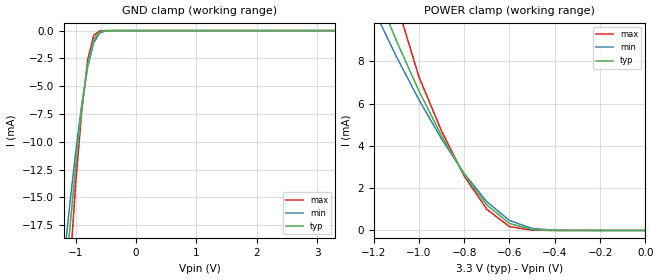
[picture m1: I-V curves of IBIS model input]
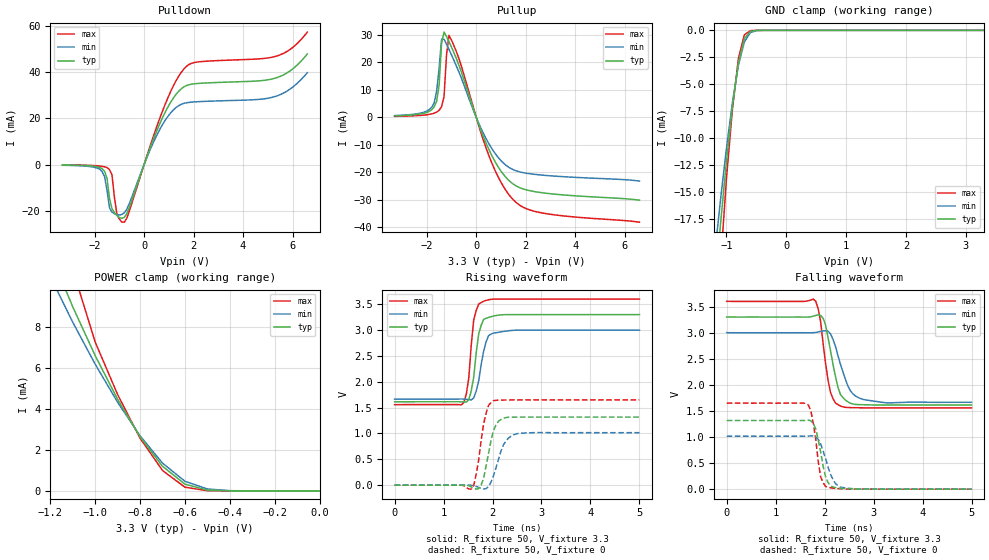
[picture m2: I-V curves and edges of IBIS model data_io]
| SOJ  Package & Industrial  operation.
[IBIS Ver]   3.2
[Comment Char]   |_char
[File name]   as7c3256a_soji.ibs
[File Rev]   1.0
[Date]   May 19, 2004 2:59:33 PM
[Source]
Alliance Semiconductor Corporation
[Notes]
This model  is for SOJ package & Industrial operation.
[Disclaimer]
Data is for modeling purpose only and is not guaranted.
This IBIS model is provided on an "AS IS" basis and Alliance Semiconductor makes
absolutely no warranty with respect to the information contained
herein.The entire risk as to quality and performance
is with the Customer. ACCORDINGLY, IN NO EVENT SHALL THE COMPANY BE
LIABLE FOR ANY DAMAGES, WHETHER IN CONTRACT OR TORT,INCLUDING ANY
LOST PROFITS OR OTHER INCIDENTAL, CONSEQUENTIAL, EXEMPLARY, OR
PUNITIVE DAMAGES ARISING OUT OF THE USE OR APPLICATION OF THE IBIS
model provided in this package.
[Copyright]
Alliance Semiconductor Corporation
| SOJ Package & Industrial  operation.
[Component]   AS7C3256A_SOJI
Si_location Pin
Timing_location Pin
[Manufacturer]   Alliance Semiconductor Corporation
[Package]
R_pkg   158.885m   88.47m   229.3m
L_pkg   7.1455nH   4.457nH   9.834nH
C_pkg   1.118pF   0.777pF   1.459pF
[Pin] signal_name   model_name
1   A14   input
2   A12   input
3   A7   input
4   A6   input
5   A5   input
6   A4   input
7   A3   input
8   A2   input
9   A1   input
10   A0   input
11   IO0   data_io
12   IO1   data_io
13   IO2   data_io
14   GND   GND
15   IO3   data_io
16   IO4   data_io
17   IO5   data_io
18   IO6   data_io
19   IO7   data_io
20   NCE   input
21   A10   input
22   NOE   input
23   A11   input
24   A9   input
25   A8   input
26   A13   input
27   NWE   input
28   VCC   POWER
| Models and submodels in the file (2): input (Input), data_io (I/O)
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[Model]   input
Model_type Input
Vinh=2V
Vinl=0.8V
C_comp   4pF   4pF   4pF
[Model Spec]
[Temperature Range] 25   85   -40
[Voltage Range]   3.3   3.0   3.6
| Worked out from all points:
|   GND clamp passes 1 mA (typ) near -0.71 V on its own axis
|   POWER clamp passes 1 mA (typ) near -0.68 V on its own axis
[GND Clamp]
-3.3V     -7.098A    -6.841A    -8.051A
-1.2V     -24.5mA    -21.03mA   -71.59mA
-1.1V     -18.08mA   -15.8mA    -21.91mA
-1V       -12.19mA   -10.98mA   -13.83mA
-900mV    -7.049mA   -6.709mA   -7.353mA
-800mV    -3.052mA   -3.264mA   -2.619mA
-700mV    -776.2uA   -1.076mA   -424.2uA
-600mV    -102uA     -214uA     -28.92uA
-500mV    -8.916uA   -29.72uA   -1.118uA
-400mV    -568.8nA   -3.277uA   -28.76nA
3.3V      81.27pA    1.281uA    71.95pA
[POWER Clamp]
-3.3V     7.097A     6.84A      8.051A
-1.2V     11.62mA    10.47mA    61.3mA
-1.1V     8.99mA     8.237mA    10.82mA
-1V       6.605mA    6.189mA    7.271mA
-900mV    4.474mA    4.328mA    4.704mA
-800mV    2.643mA    2.691mA    2.576mA
-700mV    1.205mA    1.359mA    1.001mA
-600mV    329.9uA    471.6uA    181.9uA
-500mV    42.94uA    94.79uA    11.57uA
-400mV    3.493uA    12.38uA    421.4nA
0V        81.27pA    182.3pA    86.4pA
[Model]   data_io
Model_type I/O
Enable Active-High
Polarity Non-Inverting
Vinh=2V
Vinl=0.8V
Vref=1.72V
Vmeas=1.5V
Rref=168
Cref=30pF
C_comp   4pF   4pF   4pF
[Temperature Range] 25   85   -40
[Voltage Range]   3.3   3.0   3.6
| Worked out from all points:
|   slope of the pulldown table from 0 to 0.495 V, typ, clamps not added: 34.8 ohm
|   slope of the pullup table from 0 to 0.495 V, typ, clamps not added: 43.5 ohm
|   GND clamp passes 1 mA (typ) near -0.71 V on its own axis
|   POWER clamp passes 1 mA (typ) near -0.68 V on its own axis
|   falling waveform, R_fixture 50, V_fixture 3.3: 20-80 % time 216ps typ, 278ps min, 176ps max; typ from 3.3 V to 1.61 V
|   falling waveform, R_fixture 50, V_fixture 0: 20-80 % time 170ps typ, 221ps min, 146ps max; typ from 1.32 V to 0.002 V
|   rising waveform, R_fixture 50, V_fixture 3.3: 20-80 % time 139ps typ, 163ps min, 117ps max; typ from 1.61 V to 3.3 V
|   rising waveform, R_fixture 50, V_fixture 0: 20-80 % time 173ps typ, 219ps min, 162ps max; typ from 0 V to 1.32 V
[Pullup]
-3.3V     516uA      622uA      336uA
-1.7V     3.769mA    5.223mA    1.492mA
-1.5V     11.74mA    17.82mA    2.553mA
-1.4V     26.97mA    28.44mA    3.878mA
-1.3V     31.02mA    28.43mA    7.645mA
-1.2V     29.41mA    26.61mA    22.73mA
-1.1V     27.53mA    24.68mA    29.81mA
-700mV    18.98mA    16.5mA     21.37mA
400mV     -9.463mA   -7.81mA    -11.2mA
1.5V      -24.34mA   -19.1mA    -30.04mA
2.7V      -27.52mA   -21.09mA   -34.89mA
6.6V      -30.19mA   -23.22mA   -38.2mA
[Pulldown]
-3.3V     -217uA     -326uA     -165uA
-1.8V     -1.271mA   -2.012mA   -648uA
-1.6V     -2.883mA   -5.254mA   -991uA
-1.5V     -6.034mA   -11.2mA    -1.331mA
-1.4V     -14.8mA    -18.82mA   -2.206mA
-1.3V     -19.17mA   -20.68mA   -4.516mA
-1.1V     -22.18mA   -21.81mA   -21.61mA
-800mV    -22.95mA   -20.95mA   -25.06mA
700mV     19.32mA    16.52mA    22.02mA
1.7V      34.25mA    26.8mA     42.54mA
5.2V      37.23mA    29.25mA    46.69mA
6.6V      48.06mA    39.88mA    57.54mA
[GND Clamp]
-3.3V     -7.098A    -6.841A    -8.051A
-1.2V     -24.5mA    -21.03mA   -71.59mA
-1.1V     -18.08mA   -15.8mA    -21.91mA
-1V       -12.19mA   -10.98mA   -13.83mA
-900mV    -7.049mA   -6.709mA   -7.353mA
-800mV    -3.052mA   -3.264mA   -2.619mA
-700mV    -776.2uA   -1.076mA   -424.2uA
-600mV    -102uA     -214uA     -28.92uA
-500mV    -8.916uA   -29.72uA   -1.118uA
-400mV    -568.8nA   -3.277uA   -28.76nA
3.3V      81.27pA    1.281uA    71.95pA
[POWER Clamp]
-3.3V     7.097A     6.84A      8.051A
-1.2V     11.62mA    10.47mA    61.3mA
-1.1V     8.99mA     8.237mA    10.82mA
-1V       6.605mA    6.189mA    7.271mA
-900mV    4.474mA    4.328mA    4.704mA
-800mV    2.643mA    2.691mA    2.576mA
-700mV    1.205mA    1.359mA    1.001mA
-600mV    329.9uA    471.6uA    181.9uA
-500mV    42.94uA    94.79uA    11.57uA
-400mV    3.493uA    12.38uA    421.4nA
0V        81.27pA    182.3pA    86.4pA
[Falling Waveform]
R_fixture=50
V_fixture=3.3
V_fixture_min=3.0
V_fixture_max=3.6
0s        3.3V       3V         3.6V
1.818ns   3.329V     3.004V     3.602V
1.919ns   3.329V     3.024V     3.207V
1.97ns    3.275V     3.033V     2.788V
2.02ns    3.145V     3.036V     2.408V
2.121ns   2.649V     2.976V     1.852V
2.323ns   1.815V     2.398V     1.595V
2.525ns   1.649V     1.887V     1.564V
2.778ns   1.619V     1.724V     1.56V
5ns       1.614V     1.666V     1.558V
[Falling Waveform]
R_fixture=50
V_fixture=0
V_fixture_min=0
V_fixture_max=0
0s        1.317V     1.015V     1.649V
1.667ns   1.324V     1.019V     1.613V
1.717ns   1.311V     1.021V     1.512V
1.818ns   1.157V     1.004V     962.5mV
1.869ns   948.2mV    954.5mV    540.9mV
1.919ns   715.1mV    871.4mV    237mV
2.02ns    236.5mV    586.3mV    52.18mV
2.172ns   43.85mV    184.1mV    21.21mV
2.323ns   17.33mV    41.18mV    9.459mV
5ns       1.558mV    1.512mV    1.604mV
[Rising Waveform]
R_fixture=50
V_fixture=3.3
V_fixture_min=3.0
V_fixture_max=3.6
0s        1.612V     1.664V     1.557V
1.414ns   1.611V     1.666V     1.597V
1.515ns   1.654V     1.656V     2.073V
1.566ns   1.824V     1.649V     2.713V
1.616ns   2.09V      1.687V     3.203V
1.717ns   2.925V     2.016V     3.501V
1.818ns   3.205V     2.593V     3.556V
1.919ns   3.243V     2.891V     3.586V
2.222ns   3.296V     2.972V     3.598V
5ns       3.298V     2.998V     3.598V
[Rising Waveform]
R_fixture=50
V_fixture=0
V_fixture_min=0
V_fixture_max=0
0s        0V         0V         0V
1.566ns   -35.05mV   -655.9uV   -76.23mV
1.616ns   -58.28mV   -8.306mV   -7.95mV
1.667ns   -76.16mV   -24.91mV   213.8mV
1.768ns   4.515mV    -60.5mV    869.2mV
1.869ns   374.6mV    -65.74mV   1.394V
2.02ns    1.06V      182.5mV    1.635V
2.222ns   1.293V     779.3mV    1.647V
2.475ns   1.316V     989.5mV    1.649V
5ns       1.317V     1.016V     1.649V
[Ramp]
R_load=50
dV/dt_r   7.901E-1/1.719E-10   6.094E-1/2.187E-10   9.893E-1/1.573E-10
dV/dt_f   1.012E+0/2.156E-10   8.006E-1/2.708E-10   1.225E+0/1.688E-10
|[End   data_io
